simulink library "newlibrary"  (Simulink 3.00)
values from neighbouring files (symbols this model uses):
  k1 = KK(1)    [ch8_d.m]    (also in set_x4a.m = 1; za_podmodel_voz.m = 1; auto_param.m = 7500; auto_param_opt.m = 15000)
  k2 = KK(2)    [ch8_d.m]    (also in set_x4a.m = 2; za_podmodel_voz.m = 2; auto_param.m = 150000; auto_param_opt.m = 150000)
  m1 = 10    [ex12_2st.m]    (also in set_x4a.m = 1; za_podmodel_voz.m = 1; Naloga31.m = 500)

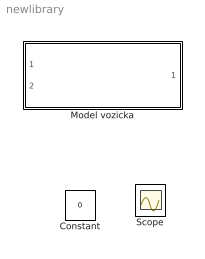
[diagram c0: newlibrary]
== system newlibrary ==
  Constant : Constant  Value=0
  Model vozicka : Subsystem  mask(Vozicek){v0=0, x0=0, m=m1, k_levo=k1, k_desno=k2}
      mask prompts: v0 "Zac. hitrost:"; x0 "Zac. odmik:"; m "Masa:"; k_levo "Konst. leve vzmeti:"; k_desno "Kons. desne vzmeti:"
      mask help: Model enega vozicka, ki se lahko povezuje z levim in desnim vozickom.
  Scope : Scope

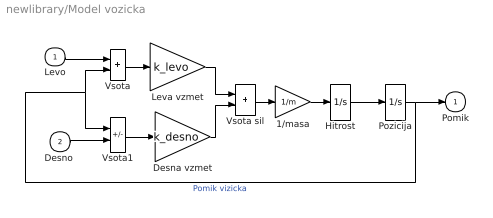
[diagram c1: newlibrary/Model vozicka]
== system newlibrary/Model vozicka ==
  Levo : Inport  Port=1  PortWidth=-1  SampleTime=-1  DataType=auto
  "Desno " : Inport  Port=2  PortWidth=-1  SampleTime=-1  DataType=auto
  1/masa : Gain  Gain=1/m  SaturateOnIntegerOverflow=on
  Desna vzmet : Gain  Gain=k_desno  SaturateOnIntegerOverflow=on
  Hitrost : Integrator  ExternalReset=none  InitialConditionSource=internal  InitialCondition=v0  LimitOutput=off  UpperSaturationLimit=inf  LowerSaturationLimit=-inf  ShowSaturationPort=off  ShowStatePort=off  AbsoluteTolerance=auto
  Leva vzmet : Gain  Gain=k_levo  SaturateOnIntegerOverflow=on
  Pozicija : Integrator  ExternalReset=none  InitialConditionSource=internal  InitialCondition=x0  LimitOutput=off  UpperSaturationLimit=inf  LowerSaturationLimit=-inf  ShowSaturationPort=off  ShowStatePort=off  AbsoluteTolerance=auto
  Vsota : Sum  Inputs=++  SaturateOnIntegerOverflow=on
  Vsota sil : Sum  Inputs=++  SaturateOnIntegerOverflow=on
  Vsota1 : Sum  Inputs=-+  SaturateOnIntegerOverflow=on
  Pomik : Outport  Port=1  InitialOutput=0
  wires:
  Pozicija/1 -> Vsota1/1, Vsota/2, Pomik/1  "Pomik vizicka"
  Hitrost/1 -> Pozicija/1
  1/masa/1 -> Hitrost/1
  Vsota sil/1 -> 1/masa/1
  Desna vzmet/1 -> Vsota sil/2
  Leva vzmet/1 -> Vsota sil/1
  Vsota/1 -> Leva vzmet/1
  Vsota1/1 -> Desna vzmet/1
  "Desno "/1 -> Vsota1/2
  Levo/1 -> Vsota/1
